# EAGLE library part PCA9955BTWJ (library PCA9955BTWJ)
NXP - PCA9955BTWJ - LED DRIVER, CONSTANT CURRENT, HTSSOP-28 Source: Datasheet
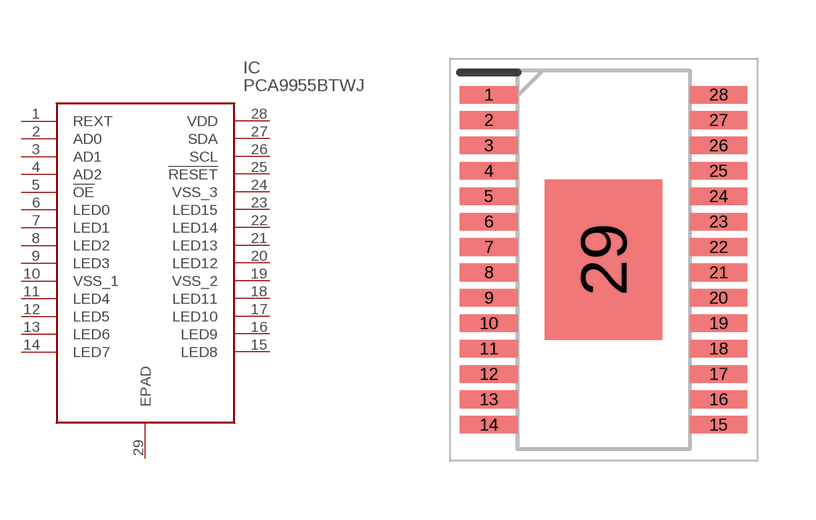
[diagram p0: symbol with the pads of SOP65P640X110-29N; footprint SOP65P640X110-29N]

Designator prefix IC

## PCA9955BTWJ (Description: NXP - PCA9955BTWJ - LED DRIVER, CONSTANT CURRENT, HTSSOP-28; Height: 1.1mm; Manufacturer_Name: NXP; Manufacturer_Part_Number: PCA9955BTWJ; Mouser_Part_Number: 771-PCA9955BTWJ; Mouser_Price-Stock: https://www.mouser.co.uk/ProductDetail/NXP-Semiconductors/PCA9955BTWJ?qs=rVFmcZtbgVjP3iVhu8%2FZog%3D%3D)  [SOP65P640X110-29N]
1  REXT  in
2  AD0  in
3  AD1  in
4  AD2  in
5  !OE  in
6  LED0  out
7  LED1  out
8  LED2  out
9  LED3  out
10  VSS_1  pwr
11  LED4  out
12  LED5  out
13  LED6  out
14  LED7  out
15  LED8  out
16  LED9  out
17  LED10  out
18  LED11  out
19  VSS_2  pwr
20  LED12  out
21  LED13  out
22  LED14  out
23  LED15  out
24  VSS_3  pwr
25  !RESET  in
26  SCL  in
27  SDA
28  VDD  pwr
29  EPAD  pwr

## Footprint SOP65P640X110-29N (pad centres in mm)
HTSSOP28
smd 1.475 x 0.45: 1 -2.938,4.225; 2 -2.938,3.575; 3 -2.938,2.925; 4 -2.938,2.275; 5 -2.938,1.625; 6 -2.938,0.975; 7 -2.938,0.325; 8 -2.938,-0.325; 9 -2.938,-0.975; 10 -2.938,-1.625; 11 -2.938,-2.275; 12 -2.938,-2.925; 13 -2.938,-3.575; 14 -2.938,-4.225; 15 2.938,-4.225; 16 2.938,-3.575; 17 2.938,-2.925; 18 2.938,-2.275; 19 2.938,-1.625; 20 2.938,-0.975; 21 2.938,-0.325; 22 2.938,0.325; 23 2.938,0.975; 24 2.938,1.625; 25 2.938,2.275; 26 2.938,2.925; 27 2.938,3.575; 28 2.938,4.225
smd 3 x 4.1: 29 0,0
